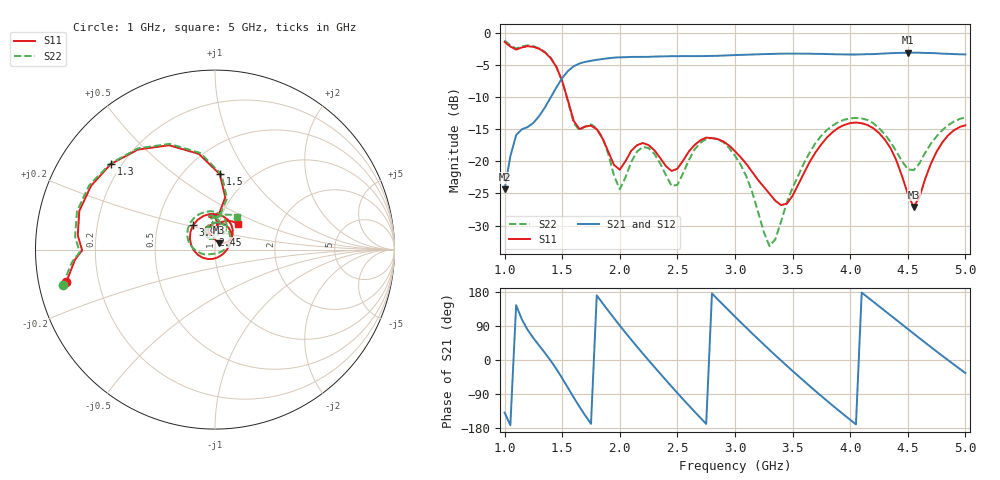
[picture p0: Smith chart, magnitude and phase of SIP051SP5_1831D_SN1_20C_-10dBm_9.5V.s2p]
# GHz  S  dB  R  50
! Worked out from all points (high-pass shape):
!   81 points, 1 GHz to 5 GHz, reference 50 ohm
!   highest |S21| = -3.10 dB at 4.5 GHz (marker M1); lowest = -24.4 dB at 1 GHz (marker M2)
!   |S21| within 3 dB of the highest: 1.543 GHz to end of sweep
!   lowest |S11| = -27.1 dB at 4.55 GHz (marker M3), VSWR 1.09, Z = 52 + j4.03 ohm
!   |S11| at or under -10 dB: 1.541 GHz to end of sweep
!   |S22| runs from -33.2 to -1.2 dB; largest |S21 - S12| = 0.002
!   S11 on the Smith chart (normalised r, x): 1 GHz: 0.08, -0.11; 1.3 GHz: 0.16, +0.35; 1.5 GHz: 0.73, +0.75; 2.45 GHz: 0.97, +0.16; 3.9 GHz: 0.76, +0.21; 5 GHz: 1.23, +0.36
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1  -1.42 -167.6  -24.37 -138.8  -24.34 -138.6  -1.20 -167.0
1.1  -2.62 -179.7  -15.93 144.8  -15.90 144.7  -2.46 -178.9
1.3  -2.49 140.6  -12.96 38.1  -12.98 38.2  -2.44 140.8
1.5  -7.52 86.3  -7.05 -48.1  -7.05 -48.1  -7.54 85.0
1.7  -14.61 100.3  -4.52 -146.6  -4.53 -146.6  -14.55 101.5
1.85  -16.44 84.5  -4.08 150.0  -4.08 150.0  -16.35 78.8
2  -21.31 107.2  -3.82 90.9  -3.81 90.9  -24.36 104.5
2.2  -17.15 104.4  -3.75 16.8  -3.75 16.9  -17.77 109.2
2.35  -19.48 88.0  -3.69 -35.7  -3.69 -35.7  -20.32 86.4
2.45  -21.51 97.0  -3.64 -70.2  -3.65 -70.2  -23.86 98.8
2.75  -16.32 85.4  -3.62 -168.6  -3.62 -168.7  -16.55 96.0
3  -18.45 38.8  -3.47 114.4  -3.47 114.5  -19.15 39.3
3.15  -21.67 14.1  -3.38 69.8  -3.38 69.9  -24.84 3.0
3.35  -26.15 -33.2  -3.27 12.5  -3.29 12.6  -32.14 -108.0
3.7  -18.59 -177.6  -3.28 -82.4  -3.28 -82.3  -17.14 169.8
3.9  -14.76 132.0  -3.36 -133.2  -3.37 -133.3  -13.87 133.6
4.1  -14.09 87.3  -3.36 177.9  -3.35 177.8  -13.34 96.5
4.35  -17.95 39.8  -3.18 117.9  -3.19 118.0  -17.01 62.3
4.5  -25.08 38.9  -3.10 81.9  -3.11 82.0  -21.24 69.1
4.55  -27.10 61.0  -3.11 70.0  -3.11 69.9  -21.39 80.9
4.8  -17.06 84.3  -3.25 10.9  -3.25 10.8  -15.16 88.2
5  -14.41 48.7  -3.37 -34.5  -3.37 -34.5  -13.16 56.6
